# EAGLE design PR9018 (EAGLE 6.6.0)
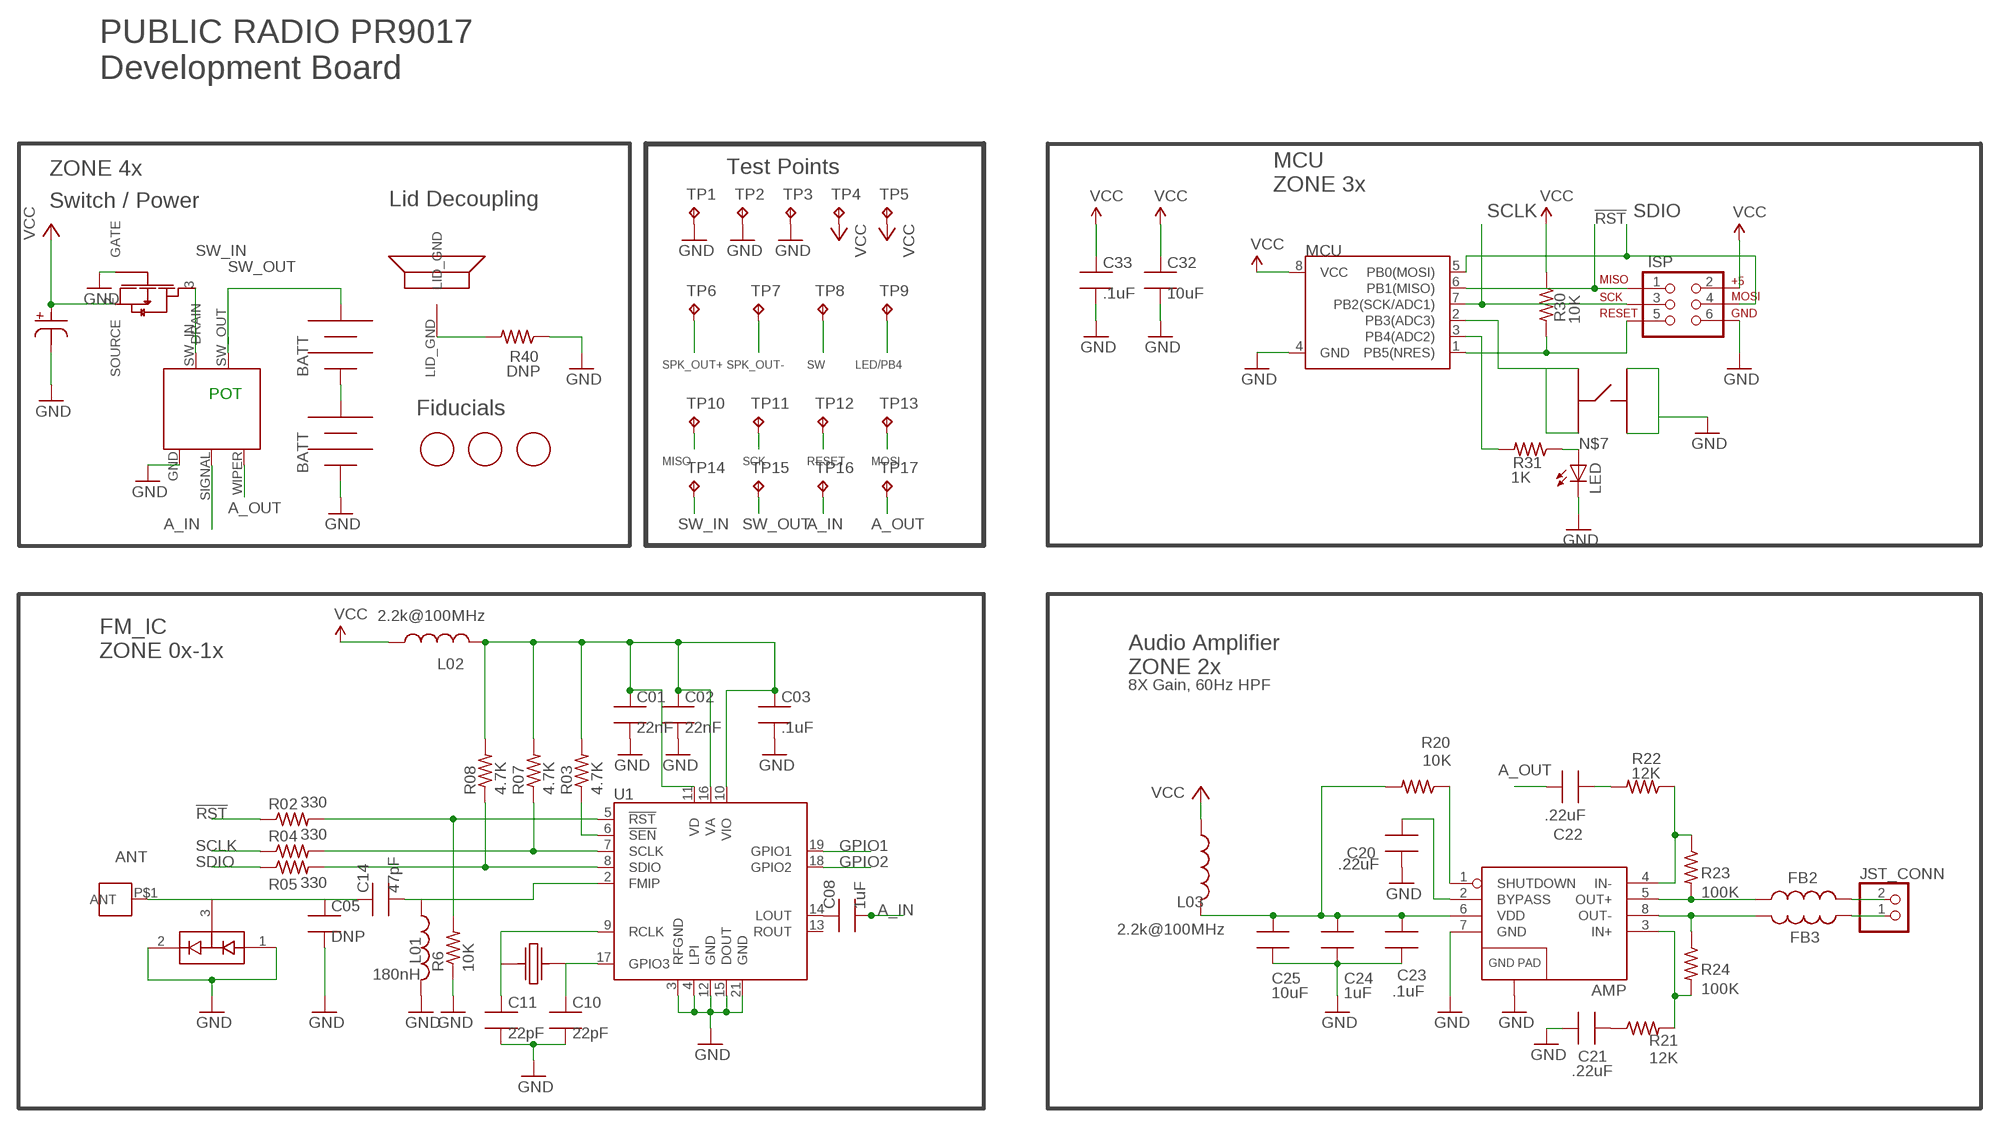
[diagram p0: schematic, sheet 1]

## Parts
AMP  TPA6203A1  [8-MSOP]
ANT_MOUNT  DNP  M3_SCREW_POST  [M3_BOLT_HOLE]
C01  22nF  C_SMT_0603_CPL  [0603_CPL]
C02  22nF  C_SMT_0603_CPL  [0603_CPL]
C03  .1uF  C_SMT_0603_CPL  [0603_CPL]
C05  DNP  C_SMT_0603_CPL  [0603_CPL]
C08  1uF  C_SMT_0603_CPL  [0603_CPL]
C10  22pF  C_SMT_0603_CPL  [0603_CPL]
C11  22pF  C_SMT_0603_CPL  [0603_CPL]
C14  47pF  C_SMT_0603_CPL  [0603_CPL]
C20  .22uF  C_SMT_0603_CPL  [0603_CPL]
C21  .22uF  C_SMT_0603_CPL  [0603_CPL]
C22  .22uF  C_SMT_0603_CPL  [0603_CPL]
C23  .1uF  C_SMT_0603_CPL  [0603_CPL]
C24  1uF  C_SMT_0603_CPL  [0603_CPL]
C25  10uF  C_SMT_0603_CPL  [0603_CPL]
C32  10uF  C_SMT_0603_CPL  [0603_CPL]
C33  .1uF  C_SMT_0603_CPL  [0603_CPL]
C40  220uF  NICHICON_SERIESUD  [NICHICON_UD_63]
D1  BAV99  [SOT23_CPL]
FB2  L_SMT_0805_ADAFRUIT  [0805_ADAFRUIT]
FB3  L_SMT_0805_ADAFRUIT  [0805_ADAFRUIT]
FET1  AO3435  [SOT23_CPL]
ISP  AVR_SPI_PRG_6NS  [2X3-NS]
JP5  BK-92_MPD_AA_BATT_CLIP  [BK92_AA_BATT]
JP6  BK-92_MPD_AA_BATT_CLIP  [BK92_AA_BATT]
JST_CONN  JST_2PIN-SMT-RA  [JST-PH-2-SMT-RA]
L01  180nH  L_SMT_0805_ADAFRUIT  [0805_ADAFRUIT]
L02  2.2k@100MHz  L_SMT_0603_CPL  [0603_CPL]
L03  2.2k@100MHz  L_SMT_0603_CPL  [0603_CPL]
LED  LED  [0603_CPL]
MARK1  FIDUCIAL  [FIDUCIAL_1MM]
MARK2  FIDUCIAL  [FIDUCIAL_1MM]
MARK3  FIDUCIAL  [FIDUCIAL_1MM]
MCU  ATTINY45TINY45-20-SMT  [8-SOIC]
R1  RV170SF_TAIWANA_POT_SW  [RV170SF_SW_POT]
R02  330  R_SMT_R0603_CPL  [0603_CPL]
R03  4.7K  R_SMT_R0603_CPL  [0603_CPL]
R04  330  R_SMT_R0603_CPL  [0603_CPL]
R05  330  R_SMT_R0603_CPL  [0603_CPL]
R6  10K  R_SMT_R0603_CPL  [0603_CPL]
R07  4.7K  R_SMT_R0603_CPL  [0603_CPL]
R08  4.7K  R_SMT_R0603_CPL  [0603_CPL]
R20  10K  R_SMT_R0603_CPL  [0603_CPL]
R21  12K  R_SMT_R0603_CPL  [0603_CPL]
R22  12K  R_SMT_R0603_CPL  [0603_CPL]
R23  100K  R_SMT_R0603_CPL  [0603_CPL]
R24  100K  R_SMT_R0603_CPL  [0603_CPL]
R30  10K  R_SMT_R0603_CPL  [0603_CPL]
R31  1K  R_SMT_R0603_CPL  [0603_CPL]
R40  DNP  R_SMT_R0603_CPL  [0603_CPL]
SPKR_PLACE  DNP  PR2023_SPKR  [PR2023_SPKR_PLACE]
SW1  C&K_PTS645  [C&K_PTS645_SMT]
TP1  TPTP20R  [TP20R]
TP2  TPTP20R  [TP20R]
TP3  TPTP20R  [TP20R]
TP4  TPTP20R  [TP20R]
TP5  TPTP20R  [TP20R]
TP6  TPTP20R  [TP20R]
TP7  TPTP20R  [TP20R]
TP8  TPTP20R  [TP20R]
TP9  TPTP20R  [TP20R]
TP10  TPTP20R  [TP20R]
TP11  TPTP20R  [TP20R]
TP12  TPTP20R  [TP20R]
TP13  TPTP20R  [TP20R]
TP14  TPTP20R  [TP20R]
TP15  TPTP20R  [TP20R]
TP16  TPTP20R  [TP20R]
TP17  TPTP20R  [TP20R]
U1  SI4702-C19-GMR  [SI470X_20_QFN]
X1  ABS25XTAL  [4-SOJ]

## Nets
3.3V: C01.1 C02.1 C03.1 L02.2 R03.2 R07.2 R08.2 U1.10(VIO) U1.11(VD) U1.16(VA)
!RST: ISP.1 MCU.6(PB1(MISO)) R02.1 TP10.TP
!RST-L: R02.2 R6.2 U1.5(!RST)
!SEN-L: R03.1 U1.6(!SEN)
A_IN: C08.2 R1.SIGNAL TP16.TP
A_OUT: C22.2 R1.WIPER TP17.TP
ANT [antenna]: ANT_MOUNT.P$1(ANT) C05.1 C14.1 D1.3(COM)
GND: AMP.7(GND) AMP.9(GND) C01.2 C02.2 C03.2 C05.2 C10.2 C11.2 C20.1 C21.1 C23.2 C24.2 C25.2 C32.2 C33.2 C40.P$2 D1.1(A1) D1.2(C2) FET1.1(GATE) ISP.6 JP6.NEG JP6.NEG@2(NEG) L01.2 LED.2(C) MCU.4(GND) R1.GND R6.1 R40.1 SW1.P$1 SW1.P$2 TP1.TP TP2.TP TP3.TP U1.3(RFGND) U1.4(LPI) U1.12(GND) U1.15(DOUT) U1.21(GND)
GPIO1: U1.19(GPIO1)
GPIO2: U1.18(GPIO2)
LED/PB4: MCU.3(PB4(ADC2)) R31.2 TP9.TP
N$1: C11.1 U1.9(RCLK) X1.P$1
N$2: AMP.6(VDD) C23.1 C24.1 C25.1 L03.2 R20.2
N$3: C22.1 R22.2
N$4: AMP.5(OUT+) FB2.1 R23.2
N$5: AMP.3(IN+) R21.2 R24.2
N$7: LED.1(A) R31.1
N$8: R40.2 SPKR_PLACE.LID_GND
N$9: C08.1 U1.14(LOUT)
N$10: C10.1 U1.17(GPIO3) X1.P$4
N$11: AMP.8(OUT-) FB3.2 R24.1
N$12: AMP.2(BYPASS) C20.2
N$13: JP5.NEG JP5.NEG@2(NEG) JP6.POS JP6.POS@2(POS)
N$14: AMP.4(IN-) R22.1 R23.1
N$16 [antenna]: C14.2 L01.1 U1.2(FMIP)
N$20: AMP.1(SHUTDOWN) R20.1
N$23: C21.2 R21.1
RESET: ISP.5 MCU.1(PB5(NRES)) R30.2 TP12.TP
SCLK: ISP.3 MCU.7(PB2(SCK/ADC1)) R04.1 TP11.TP
SCLK-L: R04.2 R07.1 U1.7(SCLK)
SDIO: ISP.4 MCU.5(PB0(MOSI)) R05.1 TP13.TP
SDIO-L: R05.2 R08.1 U1.8(SDIO)
SPK_OUT+: FB2.2 JST_CONN.2 TP6.TP
SPK_OUT-: FB3.1 JST_CONN.1 TP7.TP
SW: MCU.2(PB3(ADC3)) SW1.P$3 SW1.P$4 TP8.TP
SW_IN: FET1.3(DRAIN) R1.SW_IN TP14.TP
SW_OUT: JP5.POS JP5.POS@2(POS) R1.SW_OUT TP15.TP
VCC: C32.1 C33.1 C40.P$1 FET1.2(SOURCE) ISP.2 L02.1 L03.1 MCU.8(VCC) R30.1 TP4.TP TP5.TP
Unconnected: U1.13(ROUT)

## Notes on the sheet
- PUBLIC RADIO PR9017
  Development Board
- ZONE 4x | Test Points
- MCU
  ZONE 3x
- Switch / Power | Lid Decoupling
- POT
- Fiducials
- MISO | SCK | RESET | MOSI
- FM_IC
  ZONE 0x-1x
- Audio Amplifier 
  ZONE 2x
- 8X Gain, 60Hz HPF

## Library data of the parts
AMP = PR_Parts_Library:TPA6203A1: IC AMP AUDIO PWR 1.25W AB 8MSOP; MFG_PN: TPA6203A1DGNR
ANT_MOUNT = PR_Parts_Library:M3_SCREW_POST: Antenna mounting hole for M3 screw.; MFG_PN: DNP
C01 C02 = PR_Parts_Library:C_SMT: SMT capacitor; MFG_PN: CL10B223KB8NNNC; TOL: 10%; VOLTAGE: 16V
C03 C23 C33 = PR_Parts_Library:C_SMT: SMT capacitor; MFG_PN: CL10B104KB8SFNC; TOL: 10%; VOLTAGE: 16V
C05 = PR_Parts_Library:C_SMT: SMT capacitor; MFG_PN: DNP; TOL: 2%; VOLTAGE: 50V
C08 C24 = PR_Parts_Library:C_SMT: SMT capacitor; MFG_PN: CL10B105KP8NNNC; TOL: 10%; VOLTAGE: 10V
C10 C11 = PR_Parts_Library:C_SMT: SMT capacitor; MFG_PN: C1608C0G1H220J080AA; TOL: 5%; VOLTAGE: 50V
C14 = PR_Parts_Library:C_SMT: SMT capacitor; MFG_PN: CL10C470JB8NCNC; TOL: 5%; VOLTAGE: 50V
C20-C22 = PR_Parts_Library:C_SMT: SMT capacitor; MFG_PN: C1608X7R1C224K080AC; TOL: 10%; VOLTAGE: 16V
C25 C32 = PR_Parts_Library:C_SMT: SMT capacitor; MFG_PN: CL10A106MQ8NNNC; TOL: 20%; VOLTAGE: 6.3V
C40 = PR_Parts_Library:NICHICON_SERIESUD: Nichicon UD Series 220uf Cap; MFG_PN: UUD1C221MCL1GS; TOL: 20%; VOLTAGE: 16V
D1 = PR_Parts_Library:BAV99: DIODE ARRAY GP 100V 215MA SOT23; MFG_PN: BAV99,215
FB2 FB3 = PR_Parts_Library:L_SMT: SMT inductor; CURRENT: 2A; DCR: 45m; MFG_PN: HI0805R800R-10
FET1 = PR_Parts_Library:AO3435: MOSFET P-CH 20V 2.9A SOT23; MFG_PN: AO3435
ISP = PR_Parts_Library:AVR_SPI_PRG_6: DIL VERTICAL PC TAIL PIN HEADER; MFG_PN: M20-9980346
JP5 JP6 = PR_Parts_Library:BK-92_MPD_AA_BATT_CLIP: Thru hole AA battery clip pair.; MFG_PN: 2 of BK92
JST_CONN = PR_Parts_Library:JST_2PIN: JST 2-pin connector; MFG_PN: S2B-PH-SM4-TB(LF)(SN)
L01 = PR_Parts_Library:L_SMT: SMT inductor; CURRENT: 400mA; DCR: 640m; MFG_PN: AISC-0805-R18J-T; TOL: 5%
L02 L03 = PR_Parts_Library:L_SMT: SMT inductor; CURRENT: 150mA; DCR: 2.3; MFG_PN: HZ0603A222R-10
LED = PR_Parts_Library:LED: SMT LED; MFG_PN: LY R976-PS-36
MARK1-MARK3 = PR_Parts_Library:FIDUCIAL: 1mm fiducial.; MFG_PN: DNP
MCU = PR_Parts_Library:ATTINY45: Atmel 8-pin 2/4/8kB flash uC; MFG_PN: ATTINY45-20SUR
R1 = PR_Parts_Library:RV170SF_TAIWANA_POT_SW: Thru hole switched potentiometer.; MFG_PN: RV170SF-43-20F-A10K
R02 R04 R05 = PR_Parts_Library:R_SMT: SMT resistor; MFG_PN: MCR03ERTJ331; POWER: 1/10W; TOL: 5%
R03 R07 R08 = PR_Parts_Library:R_SMT: SMT resistor; MFG_PN: ERJ-3EKF4701V; POWER: 1/10W; TOL: 1%
R6 R20 R30 = PR_Parts_Library:R_SMT: SMT resistor; MFG_PN: ERJ-3GEYJ103V; POWER: 1/10W; TOL: 5%
R21 R22 = PR_Parts_Library:R_SMT: SMT resistor; MFG_PN: RMCF0603FT12K0; POWER: 1/10W; TOL: 1%
R23 R24 = PR_Parts_Library:R_SMT: SMT resistor; MFG_PN: RMCF0603FT100K; POWER: 1/10W; TOL: 1%
R31 = PR_Parts_Library:R_SMT: SMT resistor; MFG_PN: ERJ-3EKF1001V; POWER: 1/10W; TOL: 1%
R40 = PR_Parts_Library:R_SMT: SMT resistor; MFG_PN: ERJ-3GEY0R00V
SPKR_PLACE = PR_Parts_Library:PR2023_SPKR: Speaker placement for PR2023.; MFG_PN: DNP
SW1 = PR_Parts_Library:C&K_PTS645: SWITCH TACTILE SPST-NO 0.05A 12V; MFG_PN: PTS645SM43SMTR92 LFS
TP1-TP17 = PR_Parts_Library:TP: Test pad; MFG_PN: DNP
U1 = PR_Parts_Library:SI4702-C19-GMR: IC FM RADIO TUNER 20-QFN; MFG_PN: Si4702 C19 GMR
X1 = PR_Parts_Library:ABS25XTAL: 4PIN 32.768 Xtal; MFG_PN: ABS25-32.768KHZ-T

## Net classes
1 antenna: clearance 1.27 mm

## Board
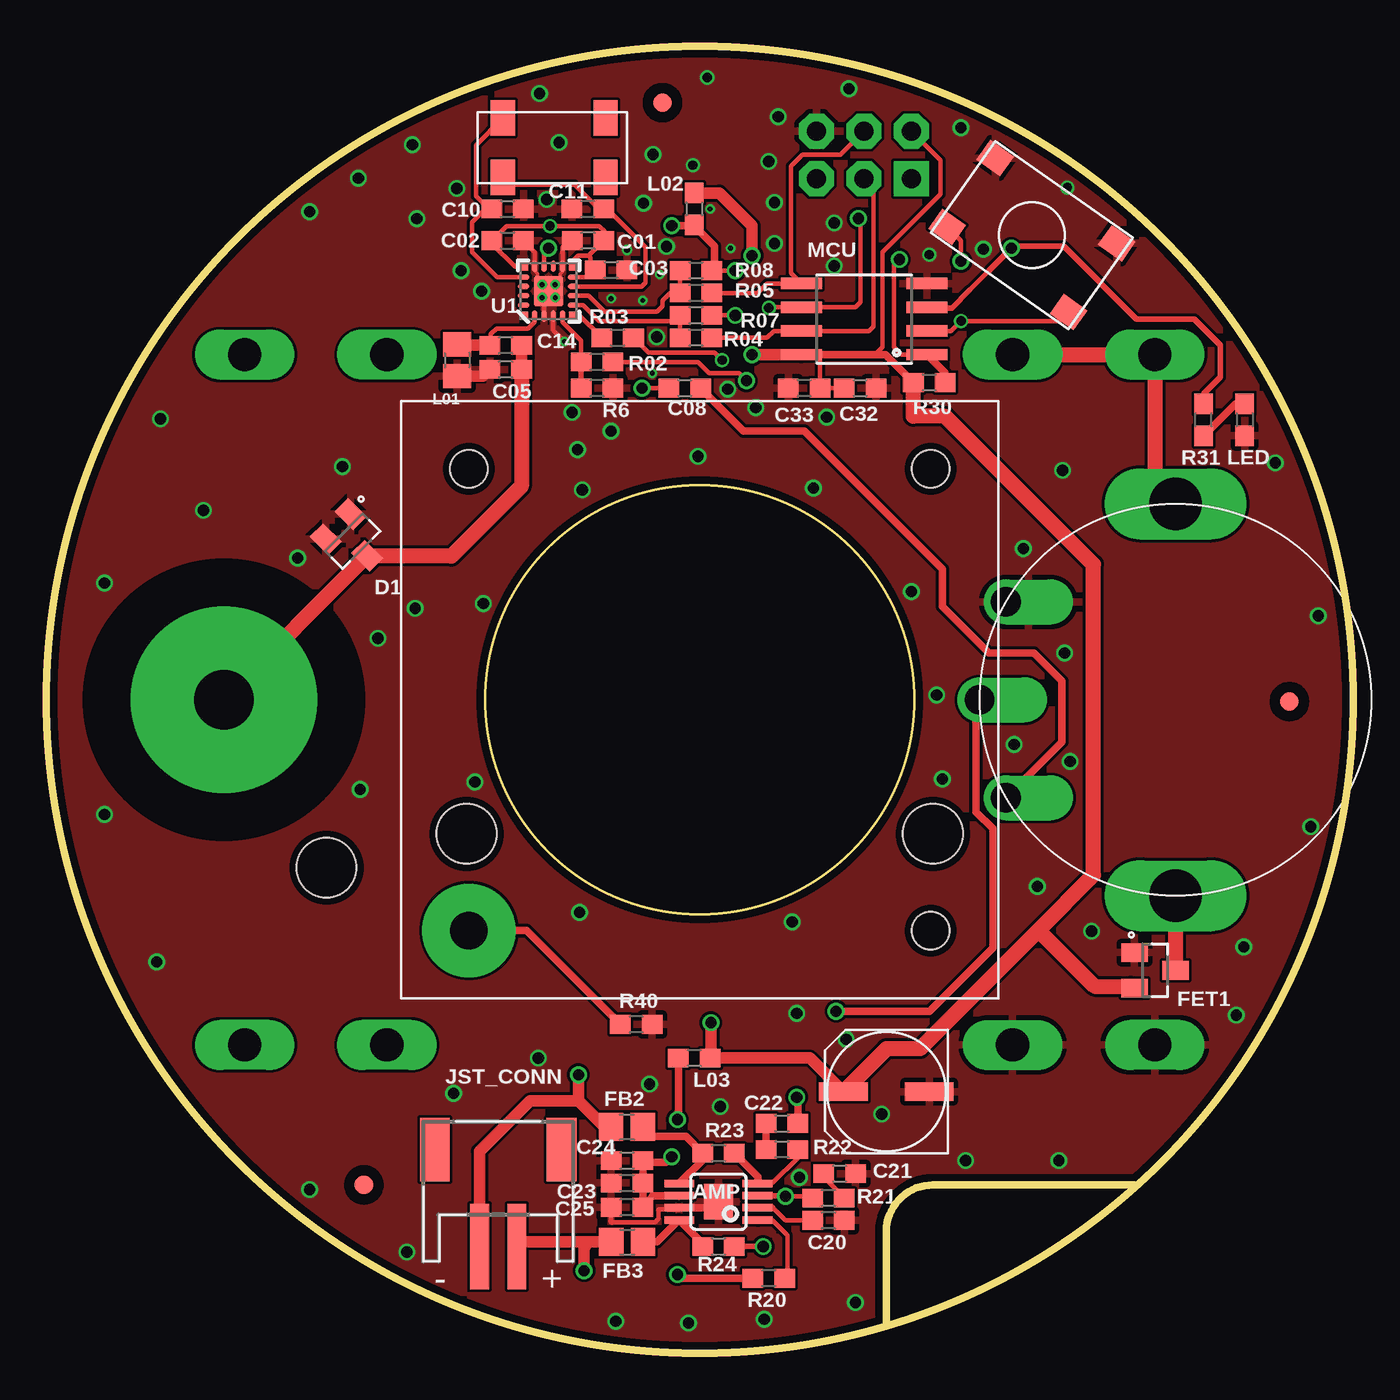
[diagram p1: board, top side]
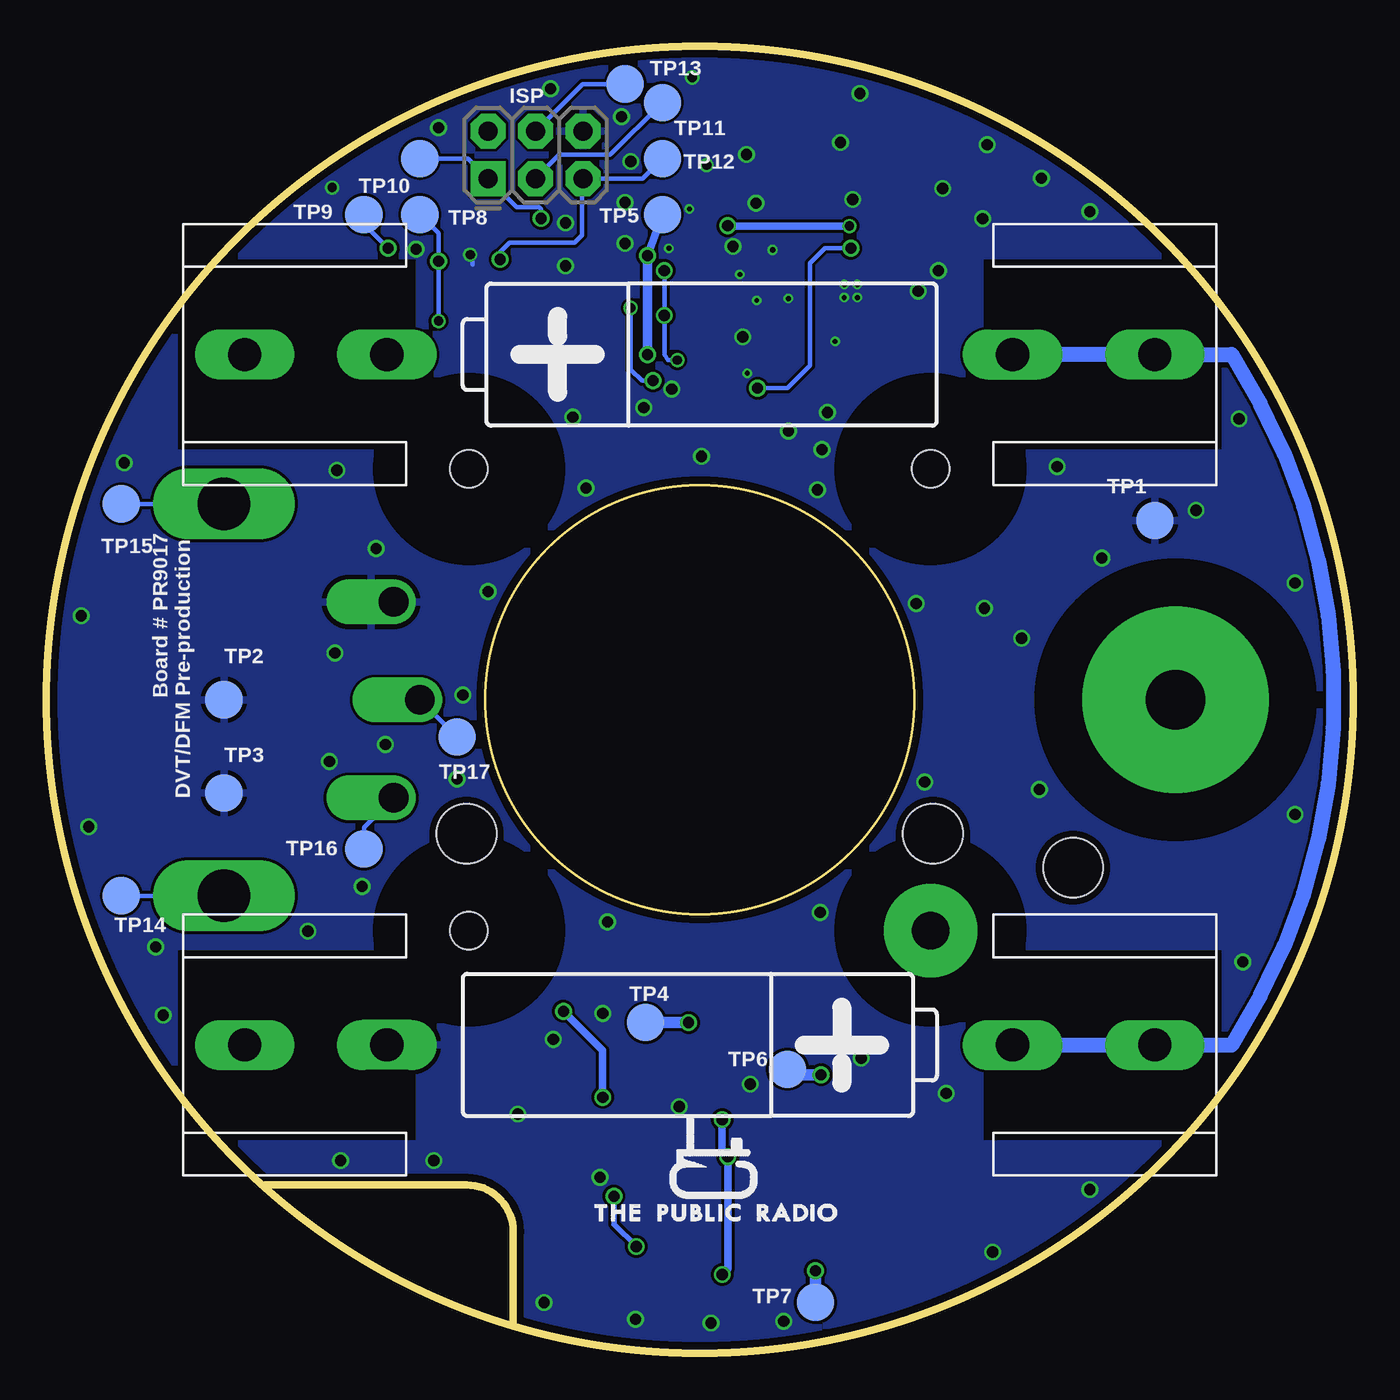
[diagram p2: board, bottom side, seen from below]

Size 70 x 70 mm. Coordinates in mm from the lower left corner, seen from the top.
Outline: 45,1.5 45,6.5 arc-90 47.5,9 58.3,9
Outline: circle at 35,35 radius 35
Copper layers (1*16): Top 0.0356mm / dielectric 1.5011mm / Bottom 0.0356mm
Design rules "LaenPCBOrder *": minimum track width 6mil, minimum drill 13mil, track to track 6mil, track to pad 6mil, pad to pad 6mil, via to via 6mil, smd to smd 6mil, copper to edge 15mil, drill to drill 6mil, minimum pad ring 7mil, minimum via ring 5mil, stop-mask expansion 3mil, vias tented up to drill 0mil, thermal gap 10mil
Holes 3.2 mm at 15,26
tRestrict: area 26.1,56.1 to 27.7,57.7; 8 lines

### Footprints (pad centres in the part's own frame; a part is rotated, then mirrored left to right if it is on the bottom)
8-MSOP = smd 0.4 x 1.6: 1 -0.975,-2.1; 2 -0.325,-2.1; 3 0.325,-2.1; 4 0.975,-2.1; 5 0.975,2.1; 6 0.325,2.1; 7 -0.325,2.1; 8 -0.975,2.1 | smd 1.89 x 1.57: 9 0,0
M3_BOLT_HOLE = drill 3.2 pad 10: P$1 0,0
0603_CPL = smd 1.1 x 1: 1 -0.85,0; 2 0.85,0
NICHICON_UD_63 = smd 1 x 2.6: P$1 0,2.3; P$2 0,-2.3
SOT23_CPL = smd 1.4 x 1: 1 -1.1,0.95; 2 -1.1,-0.95; 3 1.1,0
0805_ADAFRUIT = smd 1.3 x 1.5: 1 -0.85,0; 2 0.85,0
2X3-NS = drill 1.016 pad 1.88 square: 1 -2.54,-1.27 | drill 1.016 pad 1.88 octagon: 2 -2.54,1.27; 3 0,-1.27; 4 0,1.27; 5 2.54,-1.27; 6 2.54,1.27
BK92_AA_BATT = drill 1.778 long: NEG -24.384,0; NEG@2 -16.764,0; POS 16.764,0; POS@2 24.384,0
JST-PH-2-SMT-RA = smd 1 x 4.6: 1 1,-3.7; 2 -1,-3.7 | smd 1.6 x 3.4: NC1 -3.4,1.5; NC2 3.4,1.5
FIDUCIAL_1MM = smd 1 x 1: 1 0,0
8-SOIC = smd 0.61 x 2.21: 1 -1.905,-3.378; 2 -0.635,-3.378; 3 0.635,-3.378; 4 1.905,-3.378; 5 1.905,3.353; 6 0.635,3.353; 7 -0.635,3.353; 8 -1.905,3.353
RV170SF_SW_POT = drill 1.6 offset: GND -5.25,-9.09; SIGNAL 5.25,-9.09; WIPER 0,-10.5 | drill 2.8 long: SW_IN 10.5,0; SW_OUT -10.5,0
PR2023_SPKR_PLACE = drill 2 pad 5: LID_GND -12.37,-12.37 | hole 2: -12.37,12.37; 12.37,12.37; 12.37,-12.37 | hole 3.2: -12.497,-7.188; 12.497,-7.188
C&K_PTS645_SMT = smd 1.55 x 1.3: P$1 -3.975,2.25; P$2 3.975,2.25; P$3 -3.975,-2.25; P$4 3.975,-2.25
TP20R = smd 2 x 2: TP 0,0
SI470X_20_QFN = smd 0.34 x 0.34: 1 -1.275,1.265; 6 -1.265,-1.265; 11 1.265,-1.265; 16 1.265,1.265 | smd 0.61 x 0.28: 2 -1.335,0.75; 3 -1.335,0.25; 4 -1.335,-0.25; 5 -1.335,-0.75; 12 1.335,-0.75; 13 1.335,-0.25; 14 1.335,0.25; 15 1.335,0.75 | smd 0.28 x 0.61: 7 -0.75,-1.335; 8 -0.25,-1.335; 9 0.25,-1.335; 10 0.75,-1.335; 17 0.75,1.335; 18 0.25,1.335; 19 -0.25,1.335; 20 -0.75,1.335 | smd 1.6 x 1.6: 21 0,0
4-SOJ = smd 1.3 x 1.9: P$1 -2.75,-1.6; P$2 2.75,-1.6; P$3 2.75,1.6; P$4 -2.75,1.6

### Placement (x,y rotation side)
AMP  36,8.1 90 top
ANT_MOUNT  9.5,35 0 top
C01  29.01,59.6 180 top
C02  24.7,59.6 0 top
C03  30.24,58.03 0 top
C05  24.6,52.7 180 top
C08  34.2,51.7 0 top
C10  24.7,61.3 0 top
C11  29,61.3 180 top
C14  24.6,54 180 top
C20  41.9,7.1 180 top
C21  42.5,9.6 180 top
C22  39.4,12.3 0 top
C23  31.1,9.1 180 top
C24  31.1,10.3 180 top
C25  31.1,7.8 180 top
C32  43.6,51.7 0 top
C33  40.6,51.7 180 top
C40  45,14 90 top
D1  16.4,43.5 315 top
FB2  31.1,12.1 180 top
FB3  31.11,5.94 0 top
FET1  59.4,20.5 0 top
ISP  43.8,64.2 0 bottom
JP5  35,53.5 180 bottom
JP6  35,16.5 0 bottom
JST_CONN  24.2,9.4 0 top
L01  22,53.2 270 top
L02  34.7,61.3 270 top
L03  34.7,15.8 180 top
LED  64.2,50 270 top
MARK1  17,9 0 top
MARK2  33,67 0 top
MARK3  66.6,34.9 0 top
MCU  43.8,55.4 90 top
R1  60.5,35 270 top
R02  29.5,53.1 180 top
R03  30.6,54.4 0 top
R04  34.8,54.4 180 top
R05  34.8,56.8 180 top
R6  29.5,51.7 180 top
R07  34.8,55.6 0 top
R08  34.8,58 0 top
R20  38.7,4 180 top
R21  41.9,8.3 180 top
R22  39.4,10.9 180 top
R23  36,10.7 180 top
R24  36,5.7 0 top
R30  47.3,52 0 top
R31  62,50 90 top
R40  31.6,17.6 180 top
SPKR_PLACE  35,35 0 top
SW1  52.8,59.9 325 top
TP1  10.6,44.6 0 bottom
TP2  60.5,35 0 bottom
TP3  60.5,30 0 bottom
TP4  37.9,17.7 0 bottom
TP5  37,61 0 bottom
TP6  30.3,15.2 0 bottom
TP7  28.8,2.7 0 bottom
TP8  50,61 0 bottom
TP9  53,61 0 bottom
TP10  50,64 0 bottom
TP11  37,67 0 bottom
TP12  37,64 0 bottom
TP13  39,68 0 bottom
TP14  66,24.5 0 bottom
TP15  66,45.5 0 bottom
TP16  53,27 0 bottom
TP17  48,33 0 bottom
U1  26.9,56.9 90 top
X1  27.2,64.58 0 top

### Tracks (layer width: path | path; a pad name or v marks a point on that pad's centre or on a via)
3.3V  (via drill 0.5, 0.6)
  Top 0.254: R07.2 v36.9,55.6 | 25.23,58.16 U1.16 25.6,58.2 25.1,58.2 23.85,59.45 C02.1 24.64,60.39 v26.98,60.39 29.61,60.39 29.9,60.1 29.9,59.64 C01.1 | v36.2,53.2 35.8,53.6 32.25,53.6 R03.2 | U1.10 28.35,57.65 | R08.2 v36.9,58 | U1.11 28.16,58.48 28.47,58.79 29.05,58.79 | 29.05,58.79 C01.1 | 29.8,59.66 C01.1 | U1.10 29.07,57.65 C03.1 | U1.10 28.93,57.65 29.16,57.88 29.16,58.68 29.05,58.79
  Top 0.406: 34.7,60.4 35.8,59.3 35.8,58.05 | v33.5,60.4 34.65,60.4 L02.2
  Top 0.61: L02.2 34.7,60.4 | 35.8,58.05 R08.2
  Bottom 0.254: v36.9,58 v36.9,55.6 36.9,53.5 36.7,53.2 v36.2,53.2
  Bottom 0.406: v26.98,60.39 v33.49,60.39 v33.5,60.4
!RST  (via drill 0.5, 0.6)
  Top 0.254: 41,56.03 MCU.6 38.73,56.03 v38.7,56 | 41,56.03 43.34,56.03 43.6,56.3 43.6,60.7 v43.5,60.8 | 40.97,56 41,56.03 | R02.1 34.9,53.1 35.5,52.5 37.1,52.5 v37.5,52.1
  Bottom 0.254: v43.5,60.8 43.5,61.3 43.6,61.4 44.81,61.4 ISP.1 47.41,64 TP10.TP | v38.7,56 38.7,52.7 38.1,52.1 v37.5,52.1
!RST-L
  Top 0.254: U1.5 27.65,55.25 28.65,54.25 R02.2
  Top 0.305: R6.2 R02.2
!SEN-L
  Top 0.254: R03.1 28.52,55.63 U1.6
A_IN
  Top 0.406: R1.SIGNAL 54.4,32.74 54.4,36 52.9,37.5 50.5,37.5 48,40 48,42 40.6,49.4 37.35,49.4 C08.2
  Bottom 0.254: TP16.TP 53,28.16 R1.SIGNAL
A_OUT  (via drill 0.6)
  Top 0.406: R1.WIPER 49.8,34.8 49.8,29 50.7,28.1 50.7,21.7 47.3,18.3 v42.3,18.3 | v40.2,13.7 40.25,13.65 C22.2
  Bottom 0.254: TP17.TP R1.WIPER
  Bottom 0.406: v42.3,18.3 40.2,16.2 v40.2,13.7
ANT
  Top 0.61: C14.1 C05.1
  Top 0.813: ANT_MOUNT.P$1 9.5,35.04 D1.3 17.2,42.7 21.7,42.7 25.45,46.45 C05.1
GND  (via drill 0.25, 0.25 pad 0.1, 0.3, 0.5, 0.6)
  Top 0.2: U1.12 27.65,57.95 27.5,57.8 27.5,57.5 v27.25,57.25 | 26.34,57.46 v26.55,57.25 26.31,57.49 26.31,57.84 26.15,58 U1.15 | 27.15,56.44 v27.26,56.55
  Top 0.254: v27.25,57.25 U1.21 | v26.55,57.25 v26.55,57.24 26.57,57.23 | C25.2 30.25,7.05 | 30.3,7 32.6,7 32.79,7.19 32.79,7.69 32.8,7.7 33.3,7.7 | U1.15 26.15,59 C02.2 | U1.12 27.65,59.25 28,59.6 C01.2 | U1.4 27.15,54.8 v27.75,54.2 | U1.3 26.65,56.45 v26.55,56.55
  Top 0.305: AMP.9 35.67,7.78 AMP.7 33.83,7.7 33.3,7.7 | 30.25,7.05 30.3,7
  Top 0.406: AMP.7 36.08,7.78 36.1,7.8
  Top 0.61: L01.2 23.4,52.35 C05.2
  Bottom 0.254: 47.18,58.84 47.18,58.33
  other vias: 35.4,68.35 30.25,49.4 65.85,47.7 28.7,46.25 26.41,67.49 53.1,25 46.35,40.8 43.35,2.7 19.3,5.4 21.8,13.9 28.55,23.6 39.95,23.1 64.15,21.75 51.85,32.6 19.6,64.75 47.3,58.85 43,67.75 49,65.65 41.1,46.35 38.45,1.8 26.35,15.8 44.75,12.8 41.8,50.15 56,22.6 54.7,62.45 39,59.45 47.7,35.25 23.3,56.9 42.2,60.55 42.2,58.25 34.63,63.65 39,61.65 21.98,62.4 19.84,60.78 36.5,51.65 50.2,59.15 14.1,61.15 6.1,50.05 3.1,41.25 3.1,28.85 14.1,8.75 30.5,1.7 49.25,10.3 54.25,10.3 63.75,18.1 67.75,28.2 68.15,39.5 28.45,48.4 28.15,50.4 19.75,39.9 23.4,40.15 22.95,30.6 34.9,48.05 16.7,62.95 16.8,30.2 5.9,20.95 22.21,58 38,50.65 17.75,38.3 13.45,42.6 15.85,47.5 34.4,1.6 32.5,64.22 27.46,64.87 26.8,61.81 31.1,59.1 31.99,61.61 33.22,59.3 32.7,54.45 36.1,13.2 32.3,14.4 40.2,18.2 42.85,16.8 48,30.75 52.35,43.1 54.55,37.5 54.85,31.7 54.45,47.3 39.2,66.25 38.7,63.85 8.4,45.15 30.25,56.5 31.95,56.4 32.85,57.8 36.65,59.2 35.55,61.3 32.45,52.5 40.35,9.4
  pour Bottom: 0,35 arc90 35,0 arc90 70,35 arc90 35,70 arc90
  pour Top: 0,35 arc90 35,0 arc90 70,35 arc90 35,70 arc90
LED/PB4  (via drill 0.6)
  Top 0.254: 50.5,58 49.45,56.95 | 47.34,56.2 MCU.3
  Top 0.305: 50.5,58 v51.7,59.2 51.8,59.3 54.5,59.3 58.4,55.4 61.5,55.4 62.9,54 62.9,52.3 62,51.4 R31.2 | 49.45,56.95 48.5,56 47.21,56 MCU.3
  Bottom 0.254: TP9.TP 53,60.5 v51.7,59.2
N$1
  Top 0.254: X1.P$1 24.75,62.6 28.3,62.6 29.6,61.3 C11.1 | C11.1 29.7,61.3 | C11.1 30.05,61.3 32.1,59.25 32.1,57.36 31.89,57.15 U1.9
N$2  (via drill 0.6)
  Top 0.406: 33.88,8.4 AMP.6 32.48,8.43 C25.1 C23.1 C24.1 32.05,10.2 33.2,10.2 v33.5,10.5 | 33.8,12.8 v33.8,12.5 33.85,12.55 L03.2 | R20.2 34,4 v33.8,4.2
  Bottom 0.406: v33.8,12.5 33.8,10.8 v33.5,10.5 33.5,4.5 v33.8,4.2
N$3
  Top 0.406: C22.1 R22.2
N$4
  Top 0.406: AMP.5 35.15,10.32 R23.2 34.25,11.6 32.4,11.6 31.95,12.05 FB2.1
N$5  (via drill 0.6)
  Top 0.254: R21.2 40.96,8.39 v39.6,8.39 39.56,8.43 39.27,8.43
  Top 0.305: 38.12,8.4 AMP.3 39.27,8.43 | v38.4,5.7 R24.2
  Bottom 0.305: v39.6,8.39 39.6,6.9 v38.4,5.7
N$7
  Top 0.406: R31.1 63.7,50.85 LED.1
N$8
  Top 0.406: SPKR_PLACE.LID_GND 25.72,22.63 R40.2
N$9  (via drill 0.6)
  Top 0.254: U1.14 26.65,58.95 v26.9,59.2 | v31.9,51.7 C08.1
  Bottom 0.254: v31.9,51.7 30.3,51.7 29.1,52.9 29.1,58.4 28.3,59.2 v26.9,59.2
N$10
  Top 0.254: U1.17 24.15,57.65 22.8,59 22.8,60.6 23.5,61.3 C10.1 | C10.1 23.8,61.2 | X1.P$4 23,64.73 23,62 23.7,61.3 C10.1
N$11
  Top 0.406: R24.1 35.15,5.88 AMP.8 32.72,5.94 FB3.2
N$12
  Top 0.254: 38.9,7.8 39.4,7.3 39.6,7.1 C20.2
  Top 0.305: 38.9,7.8 38.12,7.8 AMP.2
N$13
  Bottom 0.813: JP6.POS JP6.POS@2 6.5,16.5 arc-66 6.5,53.5 JP5.NEG JP5.NEG@2
N$14
  Top 0.254: 38.12,9.1 38.9,9.1 40.25,10.45 R22.1
  Top 0.406: AMP.4 38.12,9.1 38.12,9.43 R23.1
N$16
  Top 0.254: U1.2 26.15,55.25 25.8,54.9 24.1,54.9 23.8,54.6 23.8,54.05 C14.2
  Top 0.61: C14.2 22.05,54 L01.1
N$20
  Top 0.254: 38.12,7.1 38.9,7.1 39.7,6.3 39.7,4.15
  Top 0.406: 38.12,7.1 AMP.1 | R20.1 39.7,4.15
N$21
  pour Bottom: 
N$23
  Top 0.254: R21.1 41.65,9.4 C21.2
  Top 0.305: 41.25,9.3 C21.2
RESET  (via drill 0.6)
  Top 0.254: MCU.1 45.8,53.49 45.4,53.9 45.4,58.3 v45.7,58.6
  Top 0.406: R30.2 48.15,52.52 MCU.1
  Bottom 0.254: v45.7,58.6 45.7,59 45.2,59.5 41.7,59.5 41.3,59.9 41.3,62.89 ISP.5 38.07,62.93 TP12.TP
SCLK
  Top 0.254: MCU.7 44.06,54.77 44.3,55 44.3,62.43 ISP.3 | 40.38,54.7 MCU.7 | MCU.7 38.97,54.77 38.6,54.4 R04.1
  Bottom 0.254: ISP.3 42.53,64.2 39.8,64.2 TP11.TP
SCLK-L
  Top 0.254: R04.2 R07.1 33.65,55.3 29.6,55.3 28.75,56.15 U1.7
SDIO
  Top 0.254: ISP.4 42.53,64.2 40.5,64.2 39.9,63.6 39.9,57.85 MCU.5 38.6,57.3 38.1,56.8 R05.1
  Bottom 0.254: TP13.TP 41.27,68 ISP.4
SDIO-L
  Top 0.254: R05.2 R08.1 | 33.85,57 R05.2 | R05.2 33.4,56.8 33,56.4 33,56.1 32.7,55.8 29.9,55.8 29.05,56.65 U1.8
SPK_OUT+  (via drill 0.6)
  Top 0.61: FB2.2 29.9,12.1 28.5,13.5 | 28.5,13.5 25.9,13.5 23.2,10.8 JST_CONN.2 23.2,5.1 | 28.5,13.5 v28.5,14.9
  Bottom 0.61: v28.5,14.9 30,14.9 TP6.TP
SPK_OUT-  (via drill 0.6)
  Top 0.61: FB3.1 29.1,5.94 | 29.1,5.94 25.44,5.94 JST_CONN.1 | v28.8,4.4 28.8,5.64 29.1,5.94
  Bottom 0.61: TP7.TP v28.8,4.4
SW  (via drill 0.5, 0.6)
  Top 0.254: MCU.2 48.47,54.77 v49,55.3 54.29,55.3 SW1.P$4 | v49,58.5 49,59.59 SW1.P$3
  Bottom 0.254: v49,55.3 v49,58.5 49,60 TP8.TP
SW_IN
  Top 0.813: FET1.3 R1.SW_IN
  Bottom 0.254: TP14.TP R1.SW_IN
SW_OUT
  Top 0.813: JP5.POS JP5.POS@2 59.38,46.62 R1.SW_OUT
  Bottom 0.254: TP15.TP R1.SW_OUT
VCC  (via drill 0.6)
  Top 0.254: ISP.2 47.9,63.91 47.9,62.1 44.8,59 44.8,53.9 44.4,53.49 41.4,53.49 41.45,53.45 C33.1 C32.1
  Top 0.406: R30.1 44.95,53.49 41.4,53.49 MCU.8
  Top 0.61: MCU.8 v37.8,53.49 | C40.P$1 40.9,15.8 L03.1 35.6,15.85 v35.6,17.7 | L02.1 36.05,62.15 37.8,60.4 v37.8,58.8
  Top 0.813: 53.15,22.65 46.8,16.3 45,16.3 C40.P$1 | 53.15,22.65 56.1,25.6 56.1,42.25 48.15,50.2 46.45,50.2 R30.1 | 53.15,22.65 56.15,19.65 58.1,19.65 FET1.2
  Bottom 0.406: TP5.TP v37.8,58.8
  Bottom 0.5: v37.8,53.5 v37.8,58.8
  Bottom 0.61: v37.8,53.49 v37.8,53.5 | TP4.TP v35.6,17.7

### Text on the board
bNames: Board # PR9017 / DVT/DFM Pre-production

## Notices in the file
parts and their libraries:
SparkFun-Aesthetics: Licensing: CC v3.0 Share-Alike You are welcome to use this library for commercial purposes.
